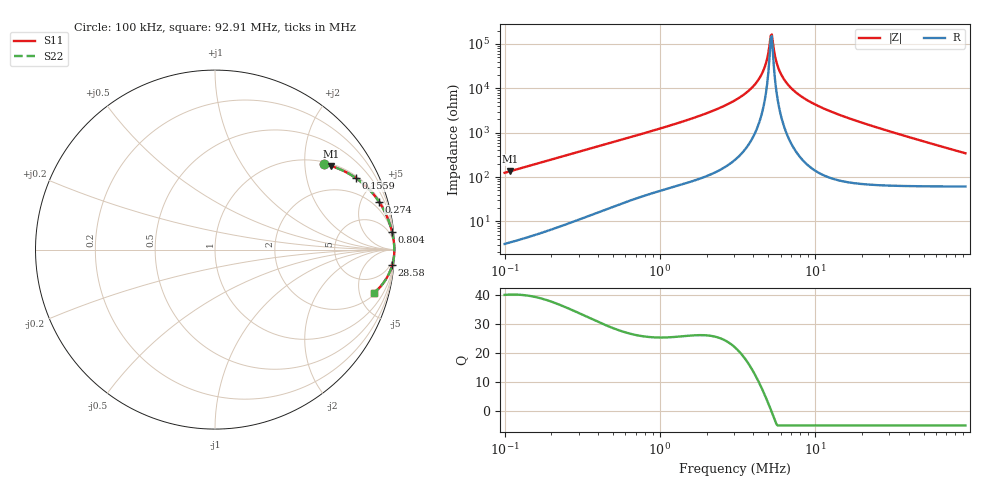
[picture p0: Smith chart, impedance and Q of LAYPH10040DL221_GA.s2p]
! LAYPH10040DL221_GA  S-PARAMETER MODEL  ( General Type )
! Model Generated by TAIYO YUDEN Corporation (http://www.ty-top.com)
! Version 1.0
! TAIYO YUDEN Control No. 180920NI43SB-FBB
! Copyright(c) 2018 TAIYO YUDEN CO.,LTD. All Rights Reserved.
! Product Description (link to TY-COMPAS)
! https://ds.yuden.co.jp/TYCOMPAS/or/detail?pn=LAYPH10040DL221MGA&u=M
! Products Name : Inductors
! Characteristics :
!  Inductance : 220 uH , SRF(min) : -Hz , DC Resistance(max) : 0.636 Ohm
!  Rated Current : Saturation :0.77 A , Temp Rise : 0.41 A (25 degC)
!  Case Size : 10.1 x 10.0 / 0.398 x 0.394 [mm/inch] , Thickness : 4 / 0.157 [mm/inch]
!  (Conditions: Temperature = 25 degC , DC Bias Current/Voltage = 0A / 0V)
! External Node Assignments :
!  1  o---GGG---o  2
! GND o---------o GND
! Frequency Range : 0.1MHz  -  92.907885MHz  [ 402 STEP ]
# MHz S RI R 50
! Freq[MHz].  S11 Real  S11 Imag  S21 Real  S21 Imag  S12 Real  S12 Imag  S22 Real  S22 Imag
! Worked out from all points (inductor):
!   401 points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, 100 kHz to 92.91 MHz, reference 50 ohm
!   read as one part in series: L = 198 uH near 103.5 kHz
!   highest Q = 40.3 at 108.9 kHz (marker M1), where L = 198 uH
!   self-resonance near 5.177 MHz
!   S11 on the Smith chart (normalised r, x): 100 kHz: 1.06, +2.49; 155.9 kHz: 1.10, +3.87; 274 kHz: 1.19, +6.77; 804 kHz: 2, +20; 28.58 MHz: 2, -23; 92.91 MHz: 2.22, -6.78
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0.1  0.6062 0.4763  0.3938 -0.4763  0.3938 -0.4763  0.6062 0.4763
0.108918  0.6448 0.4663  0.3552 -0.4663  0.3552 -0.4663  0.6448 0.4663
0.155928  0.7837 0.3993  0.2163 -0.3993  0.2163 -0.3993  0.7837 0.3993
0.274023  0.9133 0.2674  0.0867 -0.2674  0.0867 -0.2674  0.9133 0.2674
0.314158  0.9314 0.2383  0.0686 -0.2383  0.0686 -0.2383  0.9314 0.2383
0.804  0.9861 0.0992  0.0139 -0.0992  0.0139 -0.0992  0.9861 0.0992
0.986956  0.9902 0.0807  0.00978 -0.0807  0.00978 -0.0807  0.9902 0.0807
1.988488  0.9973 0.0365  0.00273 -0.0365  0.00273 -0.0365  0.9973 0.0365
3.100605  0.9989 0.0179  0.00115 -0.0179  0.00115 -0.0179  0.9989 0.0179
3.806168  0.9992 0.0106  0.000793 -0.0106  0.000793 -0.0106  0.9992 0.0106
4.363641  0.9994 0.00597  0.000649 -0.00597  0.000649 -0.00597  0.9994 0.00597
4.752802  0.9994 0.00314  0.000593 -0.00314  0.000593 -0.00314  0.9994 0.00314
5.088974  0.9994 0.000882  0.000565 -0.000882  0.000565 -0.000882  0.9994 0.000882
5.265874  0.9994 -0.000243  0.000558 0.000243  0.000558 0.000243  0.9994 -0.000243
5.356617  0.9994 -0.000806  0.000555 0.000806  0.000555 0.000806  0.9994 -0.000806
5.735498  0.9994 -0.00306  0.000555 0.00306  0.000555 0.00306  0.9994 -0.00306
6.354654  0.9994 -0.00648  0.000586 0.00648  0.000586 0.00648  0.9994 -0.00648
7.538644  0.9993 -0.0124  0.000726 0.0124  0.000726 0.0124  0.9993 -0.0124
9.575801  0.9988 -0.0213  0.00116 0.0213  0.00116 0.0213  0.9988 -0.0213
28.58008  0.9875 -0.0862  0.0125 0.0862  0.0125 0.0862  0.9875 -0.0862
30.08319  0.9862 -0.0908  0.0138 0.0908  0.0138 0.0908  0.9862 -0.0908
92.90788  0.8855 -0.2407  0.1145 0.2407  0.1145 0.2407  0.8855 -0.2407
